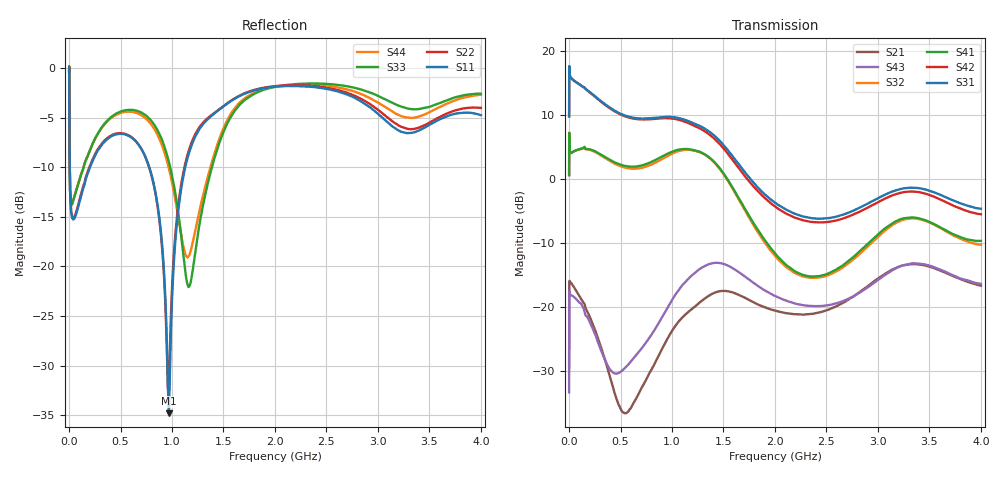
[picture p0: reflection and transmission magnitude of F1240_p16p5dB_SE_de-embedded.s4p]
! Integrated Device Technology
! Corporate Headquarters
! 6024 Silver Creek Valley Road
! San Jose, CA 95138  USA
! Phone:  1-408-284-8200
! Toll Free:  1-800-223-1366
! Webpage:  http://www.idt.com/
! Timing and RF Division
! 515 Groton Road, Suite 102
! Westford, MA 01886-6024
! Device:  F1240
! Description: Dual Intermediate Frequency Digital Variable Gain Amplifier
! Frequency:  10.0 -  500.00 MHz
! Package:  5x5 mm QFN Plastic Package: 32 pin
! Ports:  8 RF, 20 DC
!  Pin  1  = GA3 / Data  Pin 17  = RF OUT_B+
!  Pin  2  = GA4 / CLK  Pin 18  = RF OUT_B-
!  Pin  3  = GA5  Pin 19  = STBY_B
!  Pin  4  = VMODE  Pin 20  = Ground
!  Pin  5  = No Connect  Pin 21  = Ground
!  Pin  6  = GB5  Pin 22  = STB_A
!  Pin  7  = GB4  Pin 23  = RF OUT_A-  = Port 4
!  Pin  8  = GB3  Pin 24  = RF OUT_A+  = Port 3
!  Pin  9  = GB2  Pin 25  = GA0
!  Pin 10  = GB1  Pin 26  = ISET_A
!  Pin 11  = RF IN_B+  Pin 27  = VCC
!  Pin 12  = RF IN_B-  Pin 28  = Ground
!  Pin 13  = Ground  Pin 29  = RF IN_A-  = Port 2
!  Pin 14  = VCC  Pin 30  = RF IN_A+  = Port 1
!  Pin 15  = ISET_B  Pin 31  = GA1
!  Pin 16  = GB0  Pin 32  = GA2 / CSb
! Gain  = +19.5 dB
! State  = 1
! Voltage  = +5.00 V
! Current  = 85.292 mA (one channel only)
! Temperture  =  +25 C
! Test Date  =  2017-10-18
! Board  =  EB4031
! Data:  The device was measured on a custom evaluation board which has
!  individual transmission lines to the RF pins.  Data was collected
!  using a calibrated network analyzer.  The evaluation board was
!  de-embedded using Automatic Fixture Removal.
!  The reference plane is the edge of the package pin.
!  Only Channel A was measured.
!  This data is in single-ended operation.  If your needs are balanced
!  or differential S-parameters then this file needs to be used a
!  linear simulator.
! File Date:  2017-11-10  MJV
! Note:
!  Integrated Device Technology supplies this data as a sample of measured
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# Hz S dB R 100
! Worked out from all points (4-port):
!   410 points, 500 kHz to 4 GHz, reference 100 ohm
!   strongest paths, dB at 500 kHz, 930 MHz, 1.96 GHz, 2.98 GHz, 4 GHz:
!     S31: 9.8, 9.8, -3.2, -3.1, -4.6
!     S42: 9.8, 9.6, -3.8, -3.8, -5.5
!     S41: 0.6, 3.8, -10.8, -8.9, -9.7
!     S32: 0.6, 3.4, -11.2, -9.3, -10.3
!     S43: -33.4, -20.8, -17.9, -16.0, -16.4
!     S21: -29.5, -25.8, -20.4, -15.8, -16.7
!   lowest |S11| = -34.8 dB at 970 MHz (marker M1), VSWR 1.04, Z = 104 + j0.922 ohm
!   |S11| at or under -10 dB: 6.918 MHz to 203.3 MHz (196.4 MHz wide, 187 % of centre); 778.9 MHz to 1.128 GHz (349.4 MHz wide, 36.6 % of centre)
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500000  -0.30 -6.3  -29.31 12.6  -27.40 74.7  -61.81 69.1
        -29.47 12.2  -0.30 -6.3  -61.97 66.8  -27.40 75.9
        9.85 -105.4  0.65 72.5  -0.41 0.9  -33.39 -163.8
        0.64 73.6  9.83 -104.3  -33.38 -163.9  -0.42 3.2
3000000  -4.87 -53.8  -16.01 17.7  -19.76 12.3  -38.89 55.2
         -16.02 17.7  -4.83 -53.8  -38.84 55.0  -19.77 12.4
         17.25 -171.5  5.57 -4.1  -4.49 -49.2  -17.53 33.8
         5.57 -4.0  17.24 -171.3  -17.50 33.7  -4.55 -49.0
2.1e8  -9.82 -115.5  -21.85 -105.8  -22.64 -53.2  -33.73 6.7
       -21.89 -104.6  -9.65 -117.1  -33.74 6.9  -22.66 -53.1
       13.54 106.7  4.55 -58.3  -8.09 -81.8  -22.18 -113.9
       4.64 -58.3  13.49 105.9  -22.67 -112.1  -8.10 -81.1
5.6e8  -6.75 -174.7  -35.31 79.8  -24.28 -109.9  -27.69 -61.9
       -36.58 72.9  -6.70 -176.0  -27.85 -60.6  -24.44 -110.2
       9.88 20.2  1.76 -140.3  -4.23 -152.9  -29.11 77.9
       2.03 -141.3  9.76 19.1  -29.28 52.7  -4.40 -152.5
9.7e8  -34.81 14.2  -22.63 -42.2  -21.55 166.1  -23.09 -159.0
       -24.56 -47.5  -32.14 -3.6  -23.42 -154.4  -21.98 165.5
       9.76 -79.8  3.76 130.3  -9.48 145.5  -19.50 -23.6
       4.10 125.5  9.54 -81.6  -19.73 -46.4  -10.13 150.4
1.51e9  -3.78 -143.5  -17.39 162.6  -27.61 38.7  -25.01 70.1
        -17.49 167.6  -3.75 -144.1  -24.95 76.0  -28.96 36.2
        5.16 121.1  0.58 -49.8  -6.19 -123.3  -13.21 157.6
        0.68 -54.8  4.63 119.7  -13.30 150.3  -5.82 -126.9
4e9  -4.75 -157.5  -16.70 58.1  -21.74 -40.0  -19.53 -48.4
     -16.67 57.5  -4.02 -151.2  -21.99 -29.5  -25.35 -24.3
     -4.63 1.8  -10.26 -131.5  -2.59 -136.3  -15.03 89.8
     -9.66 -141.9  -5.48 10.9  -16.37 63.3  -2.69 -141.4
